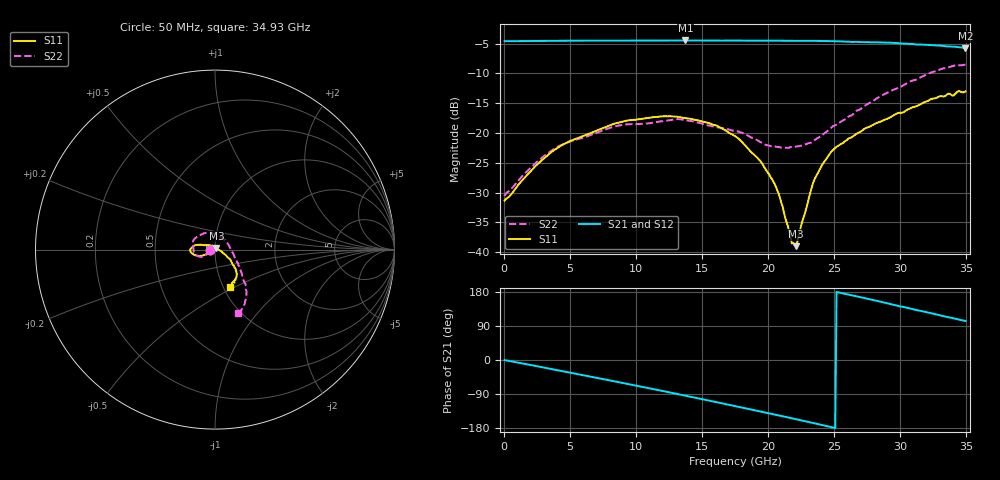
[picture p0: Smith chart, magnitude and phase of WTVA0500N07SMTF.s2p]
! 50 ohm 2-Port S-parameters measured by Modelithics Inc support@modelithics.com  Tampa, FL USA 813-866-6335 (February 2024)
! Smiths Interconnect,  5dB P/N: WTVA0500N07SMTF, Temperature: 50 C
! Board: 10 mil Rogers 4350B, Mounting Pad Dimensions: Length: 15 mils, Width: 25 mils, Gap: 40 mils.
# Hz S RI R 50
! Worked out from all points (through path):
!   352 points, 50 MHz to 34.93 GHz, reference 50 ohm
!   highest |S21| = -4.46 dB at 13.73 GHz (marker M1); lowest = -5.7 dB at 34.93 GHz (marker M2)
!   group delay of S21, straight-line fit = 20.5 ps
!   lowest |S11| = -39.0 dB at 22.09 GHz (marker M3), VSWR 1.02, Z = 50.7 + j0.849 ohm
!   |S11| at or under -10 dB: start of sweep to end of sweep
!   |S22| runs from -30.6 to -8.5 dB; largest |S21 - S12| = 0.0072
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5e7  -0.0271 -0.00051  0.5904 -0.00303  0.5898 -0.003  -0.0295 -0.00224
2.986e9  -0.0539 -0.0274  0.5601 -0.1998  0.5594 -0.2002  -0.0544 -0.0328
4.18e9  -0.0689 -0.0334  0.5271 -0.2772  0.5264 -0.277  -0.0674 -0.0392
5.8715e9  -0.0862 -0.0355  0.4619 -0.3774  0.4615 -0.3771  -0.0811 -0.0399
8.4585e9  -0.117 -0.0292  0.325 -0.5003  0.3242 -0.5001  -0.1109 -0.0268
1.1742e10  -0.1371 -0.00974  0.1051 -0.5876  0.1038 -0.5873  -0.1226 0.0226
1.3732e10  -0.1331 0.00637  -0.0434 -0.5969  -0.0441 -0.5964  -0.113 0.0605
1.612e10  -0.1129 0.0235  -0.2189 -0.5557  -0.2196 -0.5548  -0.0709 0.0864
1.7513e10  -0.0902 0.0267  -0.3144 -0.5082  -0.3145 -0.5074  -0.043 0.0946
1.94035e10  -0.0527 0.025  -0.4273 -0.4147  -0.4266 -0.4146  0.00723 0.0838
2.03985e10  -0.0307 0.0239  -0.4773 -0.356  -0.477 -0.3554  0.0276 0.0723
2.07965e10  -0.0209 0.0226  -0.4956 -0.3294  -0.4952 -0.3287  0.0364 0.0668
2.1095e10  -0.0143 0.0194  -0.5069 -0.3091  -0.5067 -0.3085  0.042 0.0627
2.17915e10  -0.000523 0.0118  -0.5333 -0.2625  -0.5332 -0.2615  0.0573 0.0505
2.209e10  0.00748 0.00836  -0.5438 -0.2409  -0.5437 -0.2394  0.0628 0.0442
2.33835e10  0.0362 -0.0102  -0.5763 -0.1427  -0.5758 -0.1426  0.0842 0.00923
2.408e10  0.0494 -0.0217  -0.5859 -0.0851  -0.5851 -0.086  0.095 -0.0114
2.51745e10  0.066 -0.0387  -0.5899 0.00443  -0.5893 0.00486  0.1092 -0.0438
2.73635e10  0.0895 -0.0634  -0.5538 0.1715  -0.5523 0.1738  0.1378 -0.1011
2.91545e10  0.1019 -0.0868  -0.4891 0.2994  -0.4857 0.3036  0.1559 -0.1574
3.23385e10  0.1201 -0.1509  -0.3013 0.4569  -0.298 0.4581  0.1727 -0.272
3.49255e10  0.0809 -0.2081  -0.1168 0.5028  -0.1163 0.5021  0.1287 -0.3528
